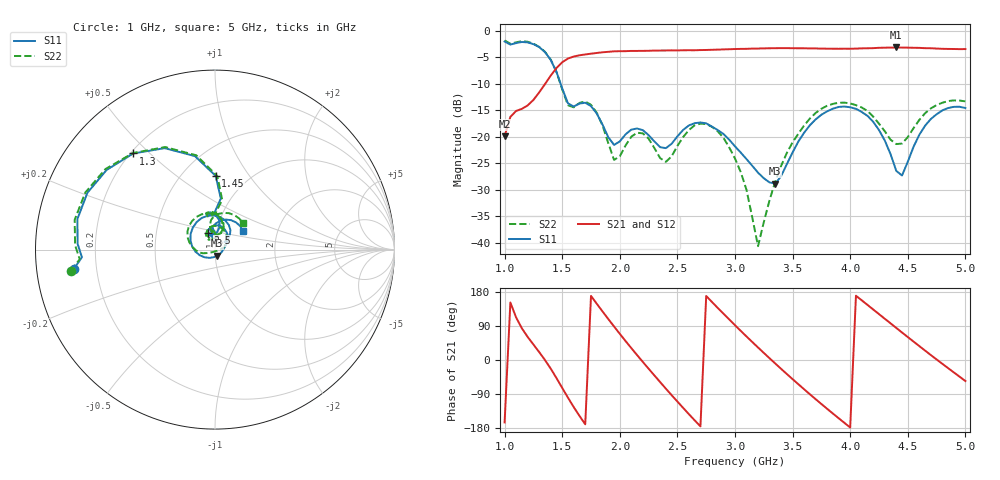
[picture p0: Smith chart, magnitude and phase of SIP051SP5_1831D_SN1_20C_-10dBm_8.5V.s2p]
# GHz  S  dB  R  50
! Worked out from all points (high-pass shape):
!   81 points, 1 GHz to 5 GHz, reference 50 ohm
!   highest |S21| = -3.14 dB at 4.4 GHz (marker M1); lowest = -19.9 dB at 1 GHz (marker M2)
!   |S21| within 3 dB of the highest: 1.491 GHz to end of sweep
!   lowest |S11| = -28.8 dB at 3.35 GHz (marker M3), VSWR 1.07, Z = 51.2 - j3.46 ohm
!   |S11| at or under -10 dB: 1.486 GHz to end of sweep
!   |S22| runs from -40.7 to -1.8 dB; largest |S21 - S12| = 0.002
!   S11 on the Smith chart (normalised r, x): 1 GHz: 0.12, -0.07; 1.3 GHz: 0.21, +0.45; 1.45 GHz: 0.72, +0.71; 2.5 GHz: 0.91, +0.17; 5 GHz: 1.33, +0.28
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1  -2.02 -172.3  -19.88 -164.8  -19.87 -164.7  -1.81 -171.7
1.15  -2.10 167.5  -14.73 83.6  -14.76 83.4  -1.95 168.0
1.3  -3.06 130.4  -11.63 21.0  -11.64 21.0  -3.02 130.3
1.45  -7.73 89.5  -7.03 -47.6  -7.01 -47.5  -7.75 88.2
1.55  -13.70 90.6  -5.23 -99.4  -5.22 -99.4  -14.05 89.7
1.7  -13.58 97.8  -4.45 -169.6  -4.46 -169.7  -13.33 97.1
1.8  -15.61 81.7  -4.17 148.4  -4.18 148.4  -15.48 77.0
1.95  -21.54 96.1  -3.87 88.4  -3.89 88.4  -24.37 89.8
2.15  -18.44 102.6  -3.79 13.0  -3.79 13.0  -19.24 105.8
2.35  -21.96 96.2  -3.71 -58.2  -3.71 -58.2  -24.05 93.0
2.5  -19.93 112.1  -3.69 -109.7  -3.68 -109.7  -21.72 125.8
2.75  -17.47 73.0  -3.61 168.9  -3.61 168.9  -17.61 81.9
3  -21.82 32.9  -3.43 91.8  -3.42 91.9  -24.11 26.8
3.2  -26.78 0.9  -3.34 33.0  -3.33 33.0  -40.67 -73.3
3.35  -28.84 -69.2  -3.27 -9.4  -3.28 -9.4  -28.43 -151.4
3.55  -20.90 -159.3  -3.28 -64.0  -3.27 -64.0  -19.42 -177.9
3.7  -16.73 159.5  -3.33 -103.3  -3.33 -103.3  -15.51 155.7
4  -14.43 91.0  -3.38 -178.2  -3.38 -178.2  -13.71 101.5
4.35  -23.26 38.8  -3.16 96.8  -3.17 96.8  -20.54 71.8
4.4  -26.45 51.0  -3.14 84.7  -3.13 84.6  -21.39 81.8
4.7  -16.64 87.7  -3.28 13.0  -3.29 13.1  -14.65 92.1
5  -14.58 33.5  -3.44 -55.6  -3.45 -55.5  -13.31 43.5
